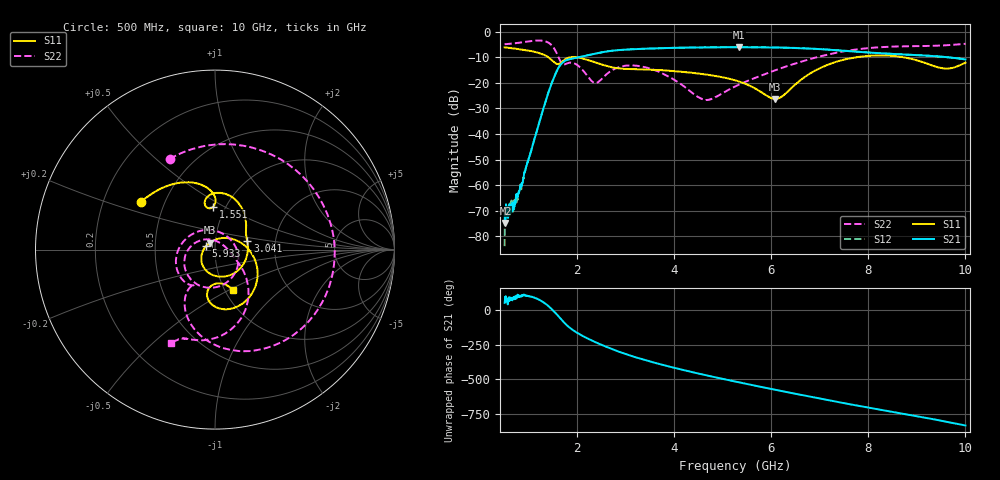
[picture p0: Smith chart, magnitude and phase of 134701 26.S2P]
!  2-Port S-parameters saved by WinCal
! VAR MeasName=S-Parameters (CALIBRATED_DATA) read from VNA (N5242A)
! VAR MeasDate=2013-7-3 16:32:37
! VAR NAME=134701 26
! VAR FILENAME=134701 26.S2P
! VAR DATE=2013-7-3 16:32:37
! VAR PHYS_PORTS=1,2
# Hz S MA R 50
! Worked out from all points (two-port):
!   1601 points, 500 MHz to 10 GHz, reference 50 ohm
!   highest |S21| = -6.09 dB at 5.327 GHz (marker M1); lowest = -74.8 dB at 517.8 MHz (marker M2)
!   |S21| within 3 dB of the highest: 2.258 GHz to 8.861 GHz (6.603 GHz wide, 119 % of centre)
!   lowest |S11| = -26.3 dB at 6.075 GHz (marker M3), VSWR 1.10, Z = 47 + j3.64 ohm
!   |S11| at or under -10 dB: 1.398 GHz to 1.881 GHz (482.6 MHz wide, 29.4 % of centre); 1.964 GHz to 7.764 GHz (5.8 GHz wide, 119 % of centre); 8.705 GHz to end of sweep
!   |S22| runs from -26.8 to -3.5 dB; largest |S21 - S12| = 0.0019
!   S11 on the Smith chart (normalised r, x): 500 MHz: 0.37, +0.25; 1.551 GHz: 0.88, +0.45; 3.041 GHz: 1.43, +0.14; 5.933 GHz: 0.90, +0.03; 10 GHz: 1.09, -0.52
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5e8  0.4913 147.5  0.0003092 51.5  6.466e-05 41.6  0.5645 116.6
5.178125e8  0.4889 146.6  0.0001825 76.9  0.0002639 79.9  0.5661 114.1
6.840625e8  0.4671 137.4  0.0003336 94.5  0.0003482 86.2  0.5859 89.4
8.621875e8  0.4441 127.1  0.001081 106.7  0.001115 106.1  0.6158 59.3
1.147188e9  0.3959 109.1  0.009995 84.4  0.009964 84.8  0.6665 0.2
1.37875e9  0.3251 93.5  0.0548 35.8  0.05498 35.6  0.6218 -60.7
1.550938e9  0.2402 92.2  0.1514 -21.7  0.1514 -21.8  0.4176 -110.7
1.770625e9  0.2952 98.6  0.2755 -106.2  0.2751 -106.2  0.2346 -121.9
2.085312e9  0.3029 69.1  0.3229 176.9  0.3226 176.9  0.1872 169.4
2.382188e9  0.2471 47.4  0.3723 125.9  0.3725 125.9  0.09893 54.2
3.04125e9  0.186 14.6  0.4459 36.1  0.446 36.2  0.217 -104.3
3.670625e9  0.1775 -28.2  0.4712 -28.7  0.4708 -28.6  0.1654 -170.7
4.626562e9  0.1458 -90.5  0.492 -109.6  0.4924 -109.7  0.04639 69.4
5.25e9  0.1118 -127.9  0.4951 -157.0  0.4956 -157.0  0.08433 -9.4
5.327188e9  0.1062 -133.0  0.4958 -162.6  0.4954 -162.7  0.09134 -13.2
5.932812e9  0.05388 159.4  0.4913 153.8  0.491 153.7  0.1554 -30.7
6.075312e9  0.04841 127.1  0.4887 143.7  0.4892 143.6  0.1746 -33.6
6.835312e9  0.1592 10.8  0.4627 90.4  0.4632 90.4  0.2961 -51.0
7.619062e9  0.2998 -40.2  0.4129 38.4  0.4135 38.3  0.4285 -73.2
8.420625e9  0.3381 -79.6  0.3684 -11.0  0.3685 -11.2  0.504 -94.8
9.554688e9  0.1898 -88.6  0.3196 -84.3  0.3198 -84.5  0.5362 -111.6
1e10  0.2467 -66.4  0.2857 -114.7  0.2853 -114.8  0.576 -115.4
